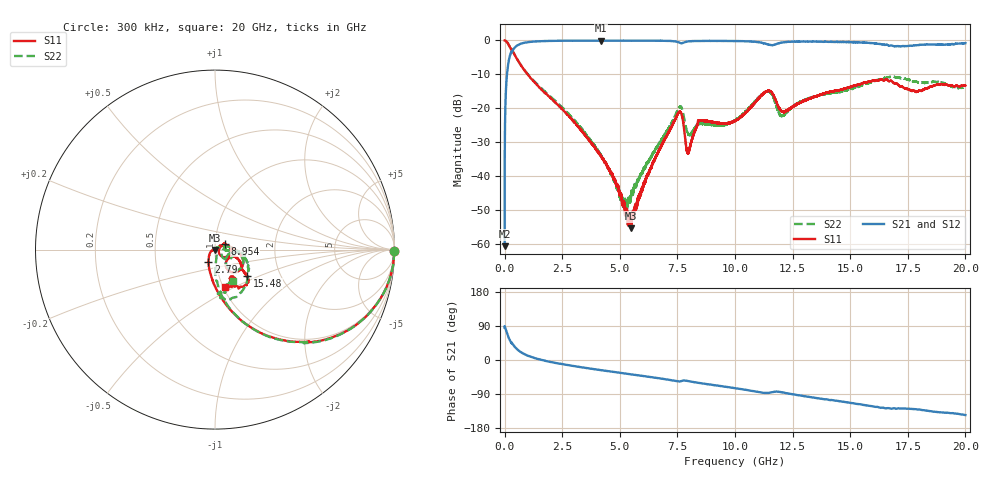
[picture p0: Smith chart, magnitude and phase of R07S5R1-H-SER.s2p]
!{R07S5R1}
!Johanson Technology Inc.
!www.johansontechnology.com
!Test Board Conditions:
!Substrate Type  RO4350B
!Substrate Thickness  10 mil
!Substrate Dk  3.66
!TL Type: GCPW
!TL Trace Width  21 mil
!TL Gap  20 mil
!Electrode orientation  Horizontal
!DUT TOPOLOGY	SERIES
!Mounting Pad LxW  16x21 mil
! Created Sat Feb  6 11:35:14 2021
# hz S ma R 50
! 2 Port Network Data from SP1.SP block
! freq  magS11  angS11  magS21  angS21  magS12  angS12  magS22  angS22
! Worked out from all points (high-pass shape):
!   20001 points, 300 kHz to 20 GHz, reference 50 ohm
!   highest |S21| = -0.05 dB at 4.182 GHz (marker M1); lowest = -60.8 dB at 300 kHz (marker M2)
!   |S21| within 3 dB of the highest: 344.8 MHz to end of sweep
!   lowest |S11| = -55.5 dB at 5.496 GHz (marker M3), VSWR 1.00, Z = 50.1 - j0.154 ohm
!   |S11| at or under -10 dB: 998.6 MHz to end of sweep
!   |S22| runs from -50.1 to 0.0 dB; largest |S21 - S12| = 0.012
!   S11 on the Smith chart (normalised r, x): 300 kHz: open; 2.79 GHz: 0.92, -0.12; 8.954 GHz: 1.11, +0.07; 15.48 GHz: 1.36, -0.42; 20 GHz: 1.02, -0.45
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300000  0.9999 -0.5  0.0009155 85.4  0.001014 86.0  0.9999 -0.5
1.113e8  0.9393 -20.6  0.3373 69.6  0.3381 69.6  0.9405 -20.6
3.033e8  0.7445 -43.3  0.6581 46.1  0.6582 46.0  0.7467 -43.4
9.833e8  0.3209 -77.9  0.9414 12.0  0.9416 12.0  0.3256 -76.7
2.7903e9  0.07626 -118.6  0.9913 -13.9  0.9909 -13.9  0.08132 -87.5
3.3343e9  0.04656 -134.2  0.9933 -19.1  0.993 -19.2  0.05028 -81.3
4.1823e9  0.01963 -159.6  0.9939 -26.8  0.9924 -26.8  0.02047 -63.2
5.2143e9  0.003549 -132.9  0.9934 -35.5  0.9925 -35.5  0.004073 0.6
5.4963e9  0.001671 -66.6  0.9917 -37.8  0.9919 -37.9  0.005268 42.5
6.6673e9  0.02223 36.8  0.9901 -47.9  0.9893 -47.9  0.02843 31.4
7.5983e9  0.08854 -5.3  0.9249 -56.5  0.9245 -56.5  0.1043 -11.7
7.9663e9  0.02193 -4.1  0.9669 -55.6  0.9669 -55.6  0.04173 -28.6
8.4463e9  0.06533 29.0  0.9825 -60.6  0.9812 -60.6  0.05901 14.2
8.9543e9  0.06337 31.8  0.9837 -65.0  0.9845 -65.1  0.05701 7.6
1.00003e10  0.06441 21.9  0.9822 -74.3  0.9814 -74.4  0.06512 -3.3
1.14023e10  0.1791 -31.3  0.8778 -87.0  0.8788 -86.9  0.1773 -30.8
1.20403e10  0.08921 -43.4  0.9348 -85.3  0.9341 -85.3  0.07721 -29.1
1.33343e10  0.1423 -22.7  0.9623 -98.4  0.9629 -98.4  0.1445 -5.5
1.54753e10  0.2296 -39.1  0.9351 -117.3  0.933 -117.4  0.2167 -29.1
1.66673e10  0.2521 -54.8  0.8399 -127.1  0.8418 -127.6  0.2873 -64.6
1.78573e10  0.1738 -59.8  0.8506 -130.1  0.8517 -130.1  0.2467 -86.4
2e10  0.2158 -74.8  0.9131 -145.2  0.9083 -145.1  0.2018 -59.8
